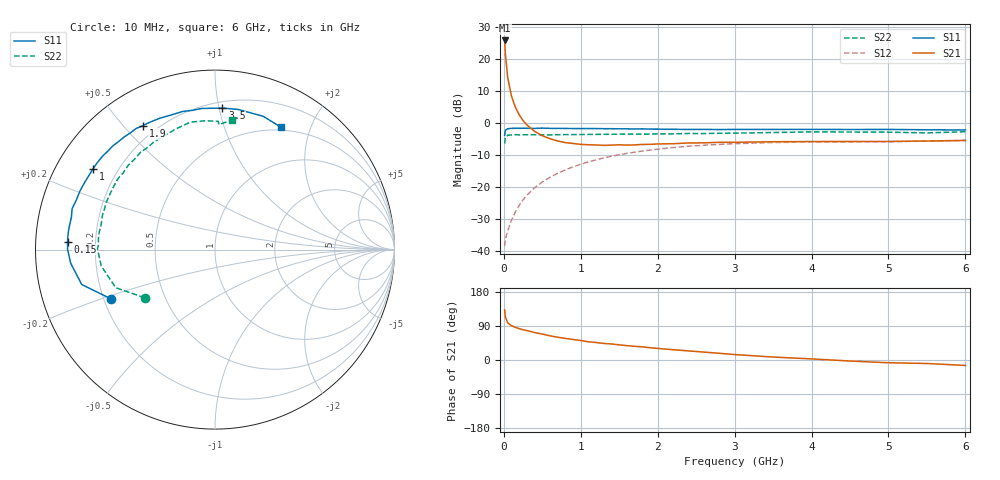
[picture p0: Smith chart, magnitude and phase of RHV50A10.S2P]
! SIEMENS Small Signal Semiconductors
! BFR106
! Si NPN RF Bipolar Junction Transistor in SOT23
! VCE = 0.5 V  IC = 100 mA
! Common Emitter S-Parameters:  August  1996
# GHz  S  MA  R  50
!  f  S11  S21  S12  S22
! GHz  MAG  ANG  MAG  ANG  MAG  ANG  MAG  ANG
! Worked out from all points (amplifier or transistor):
!   36 points, 10 MHz to 6 GHz, reference 50 ohm
!   highest |S21| = 25.7 dB at 10 MHz (marker M1)
!   |S21| within 3 dB of that: start of sweep to 17.15 MHz
!   unconditionally stable (mu >= 1): start of sweep to end of sweep
!   at 250 MHz: K = 1.89, MAG = 6.9 dB, |S12| = -23.9 dB
!   at 1.4 GHz: K = 1.30, MAG = -1.6 dB, |S12| = -10.4 dB
!   at 6 GHz: K = 1.03, MAG = -1.1 dB, |S12| = -5.5 dB
!   S11 on the Smith chart (normalised r, x): 10 MHz: 0.23, -0.21; 150 MHz: 0.10, +0.03; 1 GHz: 0.11, +0.30; 1.9 GHz: 0.15, +0.57; 3.5 GHz: 0.24, +1.02; 6 GHz: 0.46, +1.57
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0.01  0.6414 -154.7  19.19 132.2  0.012 43.4  0.4747 -145.6
0.02  0.7675 -165.3  11.84 113.5  0.0154 36.9  0.5925 -159.0
0.05  0.8076 -174.6  5.094 98.3  0.0207 46.1  0.6404 -171.8
0.1  0.8213 179.9  2.591 90.3  0.0304 57.5  0.6497 -178.1
0.15  0.8227 176.9  1.752 86.2  0.041 63.4  0.6556 179.7
0.2  0.8231 174.8  1.334 82.8  0.0518 66.7  0.6489 177.6
0.25  0.823 172.7  1.084 79.8  0.0635 68.1  0.6512 175.9
0.3  0.8218 171.0  0.927 77.6  0.0749 68.9  0.6525 174.7
0.4  0.8202 167.2  0.737 72.5  0.0976 69.1  0.6525 172.2
0.6  0.8204 160.3  0.566 63.8  0.1421 66.8  0.6497 167.5
0.8  0.8177 153.6  0.492 57.0  0.1854 63.2  0.6559 162.9
1  0.8148 146.6  0.462 51.4  0.2269 59.1  0.6576 158.4
1.1  0.8154 143.6  0.456 48.0  0.2466 57.0  0.6607 156.3
1.5  0.8069 131.7  0.455 39.9  0.3189 47.9  0.666 147.1
1.9  0.7985 120.2  0.462 32.4  0.3767 39.2  0.6694 138.2
2.2  0.794 112.9  0.473 27.2  0.4126 33.0  0.6743 131.6
2.6  0.7906 103.2  0.488 20.9  0.4481 25.3  0.6813 123.6
3.5  0.7896 87.0  0.508 7.8  0.4936 10.6  0.7064 108.2
4.5  0.7872 75.0  0.512 -2.7  0.5051 -1.8  0.7199 94.4
5  0.7898 70.1  0.513 -7.3  0.5074 -6.4  0.7152 88.6
5.5  0.7793 65.4  0.521 -9.2  0.5217 -8.7  0.6967 88.2
6  0.7741 61.8  0.531 -14.4  0.5335 -14.3  0.7276 82.7
